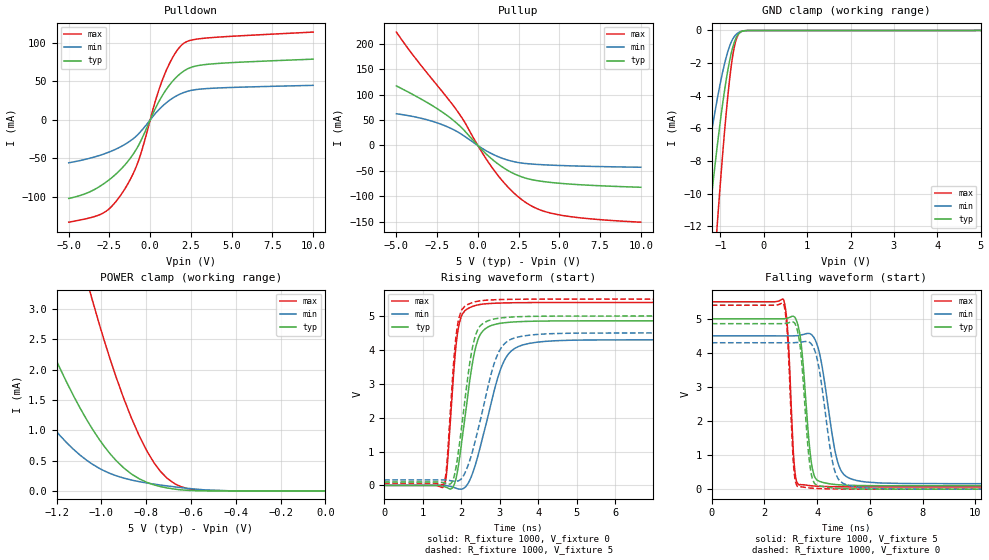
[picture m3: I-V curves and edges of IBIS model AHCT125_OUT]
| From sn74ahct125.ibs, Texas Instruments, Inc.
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[Model]   AHCT125_OUT
Model_type  3-state
Enable   Active-Low
Vref =   0
Rref =   1000
Cref =   50p
Vmeas =   1.5
| variable   typ   min   max
C_comp   2.95pF   2.40pF   3.26pF
| C_pullup   4.05pF   2.59pF   5.38pF
| C_pulldown   3.61pF   2.85pF   4.63pF
| C_tri-state   2.95pF   2.40pF   3.26pF
[Temperature Range]   40   100   -40
| Ambient temperature   25   85   -40
[Voltage range]   5   4.5   5.5
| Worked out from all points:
|   slope of the pulldown table from 0 to 0.75 V, typ, clamps not added: 23.6 ohm
|   slope of the pullup table from 0 to 0.75 V, typ, clamps not added: 31.8 ohm
|   GND clamp passes 1 mA (typ) near -0.71 V on its own axis
|   POWER clamp passes 1 mA (typ) near -1.04 V on its own axis
|   rising waveform, R_fixture 1000, V_fixture 0: 20-80 % time 360ps typ, 595ps min, 214ps max; typ from 0 V to 4.86 V
|   falling waveform, R_fixture 1000, V_fixture 5: 20-80 % time 306ps typ, 524ps min, 192ps max; typ from 5 V to 0.1 V
|   rising waveform, R_fixture 1000, V_fixture 5: 20-80 % time 346ps typ, 568ps min, 206ps max; typ from 0.1 V to 5 V
|   falling waveform, R_fixture 1000, V_fixture 0: 20-80 % time 288ps typ, 472ps min, 187ps max; typ from 4.86 V to 0 V
[GND Clamp]
| AHCT125_OUT
|   Voltage   I(typ)   I(min)   I(max)
-5V       -156.5mA   -102.6mA   -199mA
-1.56V    -19.95mA   -12.6mA    -31.6mA
-1.51V    -18.47mA   -11.64mA   -29.44mA
-1.28V    -12.08mA   -7.473mA   -19.85mA
-1.255V   -11.44mA   -7.051mA   -18.85mA
-1.08V    -7.224mA   -4.302mA   -12.14mA
-1.06V    -6.78mA    -4.014mA   -11.41mA
-885mV    -3.33mA    -1.825mA   -5.586mA
-775mV    -1.685mA   -870.1uA   -2.689mA
-675mV    -683.4uA   -355uA     -946.2uA
-555mV    -133.4uA   -88.98uA   -136uA
5V        51.2nA     8.581uA    478.9nA
[POWER Clamp]
| AHCT125_OUT
|   Voltage   I(typ)   I(min)   I(max)
-5V       76.73mA    49.29mA    123.6mA
-1.585V   6.009mA    3.217mA    12.72mA
-1.335V   3.331mA    1.637mA    7.782mA
-1.305V   3.05mA     1.477mA    7.246mA
-1.185V   2.024mA    914.1uA    5.24mA
-1.065V   1.172mA    504.1uA    3.477mA
-1.04V    1.02mA     440.6uA    3.143mA
-935mV    504.1uA    251.7uA    1.886mA
-830mV    198.2uA    152.3uA    901.8uA
-705mV    47.93uA    81.67uA    204.2uA
-580mV    4.11uA     29.95uA    18.1uA
-84.45fV  51.2nA     2.845nA    733.5nA
[Pulldown]
| AHCT125_OUT
|   Voltage   I(typ)   I(min)   I(max)
-5V       -102.3mA   -55.88mA   -133.2mA
-3.84V    -94.93mA   -50.7mA    -128.3mA
-2.855V   -83.24mA   -44.53mA   -120.9mA
-2.275V   -73.79mA   -39.74mA   -110.6mA
-1.62V    -60.27mA   -32.77mA   -92.03mA
-710mV    -32.95mA   -18.13mA   -52.68mA
335mV     15.63mA    8.704mA    25.86mA
860mV     35.56mA    19.9mA     58.01mA
1.455V    52.18mA    29.28mA    83.99mA
2.02V     62.88mA    35.23mA    99.01mA
3.59V     72.43mA    40.86mA    106.7mA
10V       78.98mA    44.89mA    114.2mA
[Pullup]
| AHCT125_OUT
|   Voltage   I(typ)   I(min)   I(max)
-5V       117mA      62.33mA    222.6mA
-3.305V   87.97mA    52.06mA    149.9mA
-1.93V    59.9mA     37.54mA    95.73mA
-945mV    33.27mA    20.92mA    52.82mA
165mV     -5.62mA    -3.532mA   -8.809mA
950mV     -29.02mA   -17.71mA   -46.65mA
1.795V    -48.11mA   -28.27mA   -79.78mA
2.64V     -61mA      -34.23mA   -104.9mA
3.64V     -68.99mA   -37.14mA   -124.1mA
4.87V     -73.75mA   -39.05mA   -135.5mA
6.86V     -78.05mA   -40.91mA   -143.8mA
10V       -82mA      -42.73mA   -150.6mA
[Ramp]
| AHCT125_OUT
| variable   typ   min   max
dV/dt_r   2.98/3.74E-10   2.65/6.12E-10   3.28/2.20E-10
dV/dt_f   2.99/3.19E-10   2.65/5.39E-10   3.31/2.02E-10
R_load = 1000
[Rising Waveform]
| AHCT125_OUT
R_fixture =   1000
C_fixture =   0
L_fixture =   0
V_fixture =   0
V_fixture_min = 0
V_fixture_max = 0
|   Time   V(typ)   V(min)   V(max)
0s        211.5pV    425.8pV    97.75pV
1.555ns   -29.72mV   -171.4uV   -20.71mV
1.635ns   -68.14mV   -10.63mV   531.8mV
1.79ns    -46.71mV   -53.94mV   3.085V
1.95ns    745.8mV    -109.5mV   4.777V
2.32ns    3.784V     437.9mV    5.292V
2.615ns   4.613V     1.674V     5.358V
3.225ns   4.812V     3.875V     5.389V
4.43ns    4.854V     4.269V     5.399V
50ns      4.858V     4.298V     5.399V
[Falling Waveform]
| AHCT125_OUT
R_fixture =   1000
C_fixture =   0
L_fixture =   0
V_fixture =   5
V_fixture_min = 4.5
V_fixture_max = 5.5
|   Time   V(typ)   V(min)   V(max)
0s        5V         4.5V       5.5V
2.72ns    5.001V     4.499V     5.57V
2.885ns   5.024V     4.499V     4.576V
3.13ns    5.059V     4.501V     711.4mV
3.31ns    4.678V     4.515V     125.4mV
3.825ns   572.6mV    4.503V     95.89mV
4.565ns   147mV      1.615V     73.19mV
5.01ns    119.9mV    430.9mV    69.26mV
6.395ns   101.7mV    181.2mV    66.14mV
50ns      99.57mV    160.9mV    65.74mV
[Rising Waveform]
| AHCT125_OUT
R_fixture =   1000
C_fixture =   0
L_fixture =   0
V_fixture =   5
V_fixture_min = 4.5
V_fixture_max = 5.5
|   Time   V(typ)   V(min)   V(max)
0s        99.57mV    160.9mV    65.74mV
1.555ns   75.72mV    160.8mV    73.91mV
1.63ns    52.15mV    153mV      656mV
1.78ns    133.7mV    129.5mV    3.238V
1.93ns    1.014V     135.9mV    4.882V
2.285ns   4.024V     969.3mV    5.392V
2.58ns    4.79V      2.332V     5.46V
3.105ns   4.952V     4.158V     5.487V
4.29ns    4.996V     4.476V     5.499V
50ns      5V         4.5V       5.5V
[Falling Waveform]
| AHCT125_OUT
R_fixture =   1000
C_fixture =   0
L_fixture =   0
V_fixture =   0
V_fixture_min = 0
V_fixture_max = 0
|   Time   V(typ)   V(min)   V(max)
0s        4.858V     4.298V     5.399V
2.715ns   4.859V     4.298V     5.458V
2.87ns    4.876V     4.298V     4.531V
3.115ns   4.895V     4.299V     588.2mV
3.33ns    4.323V     4.313V     68.39mV
3.78ns    423.2mV    4.259V     30.21mV
4.48ns    44.73mV    1.25V      8.105mV
4.89ns    20.48mV    219.9mV    4.075mV
6.26ns    2.259mV    17.48mV    493.1uV
50ns      376.1pV    -4.845nV   195.6pV
